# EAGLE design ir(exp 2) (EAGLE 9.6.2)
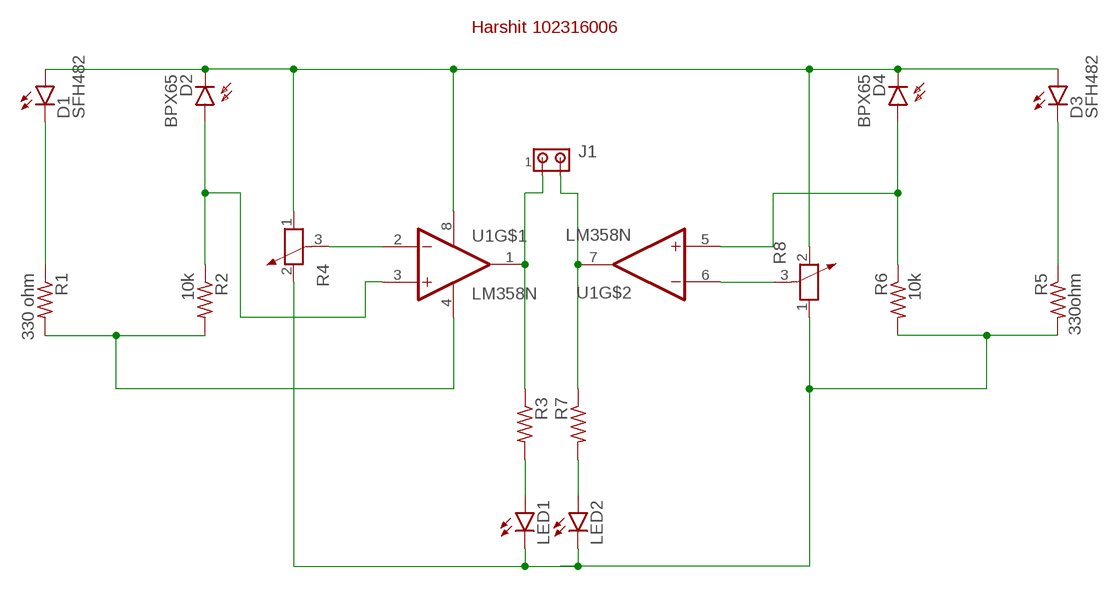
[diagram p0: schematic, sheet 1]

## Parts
D1  SFH482  [SFH482]
D2  BPX65  [BPX65]
D3  SFH482  [SFH482]
D4  BPX65  [BPX65]
J1  MTA02-100  [10X02MTA]
LED1  LED3MM  [LED3MM]
LED2  LED3MM  [LED3MM]
R1  330 ohm  R-US_0204/5  [0204/5]
R2  10k  R-US_0204/5  [0204/5]
R3  R-US_0204/5  [0204/5]
R4  POTENTIOMETER_PT-10  [PT-10]
R5  330ohm  R-US_0204/5  [0204/5]
R6  10k  R-US_0204/5  [0204/5]
R7  R-US_0204/5  [0204/5]
R8  POTENTIOMETER_PT-10  [PT-10]
U1  LM358N  [DIP762W46P254L960H508Q8]

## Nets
N$1: R8.3 U1.6(2IN-)
N$2: D1.K(C) R1.1
N$3: R1.2 R2.2 U1.4(GND)
N$4: D2.A R2.1 U1.3(1IN+)
N$6: LED1.A R3.2
N$7: J1.1 R3.1 U1.1(1OUT)
N$8: R4.3 U1.2(1IN-)
N$9: D1.A D2.K(C) D3.A D4.K(C) R4.1 R8.2 U1.8(VCC)
N$10: D3.K(C) R5.1
N$11: LED1.K(C) LED2.K(C) R4.2 R5.2 R6.2 R8.1
N$12: D4.A R6.1 U1.5(2IN+)
N$14: J1.2 R7.1 U1.7(2OUT)
N$15: LED2.A R7.2

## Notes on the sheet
- Harshit 102316006

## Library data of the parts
D1 D3 = led:SFH482: IR LED
D2 D4 = opto-trans-siemens:BPX65: PHOTO DIODE; MPN: BPX65.; OC_FARNELL: 327451; OC_NEWARK: 06WX2764
J1 = con-amp:MTA02-100: AMP connector
LED1 LED2 = led:LED: LED
R1-R3 R5-R7 = rcl:R-US_: RESISTOR, American symbol; SPICEPREFIX: R
R4 R8 = rcl:POTENTIOMETER_: Potentiometer; SPICEMODEL: POT; SPICEPREFIX: X
U1 = LM358N:LM358N: IC OPAMP GP 2 CIRCUIT 8DIP Check availability; AVAILABILITY: Not in stock; CHECK_PRICES: https://www.snapeda.com/parts/LM358N/Harris/view-part/?ref=eda; DESCRIPTION: General Purpose Amplifier 2 Circuit 8-PDIP; MF: Harris Corporation; MP: LM358N; PACKAGE: None; PRICE: None; SNAPEDA_LINK: https://www.snapeda.com/parts/LM358N/Harris/view-part/?ref=snap

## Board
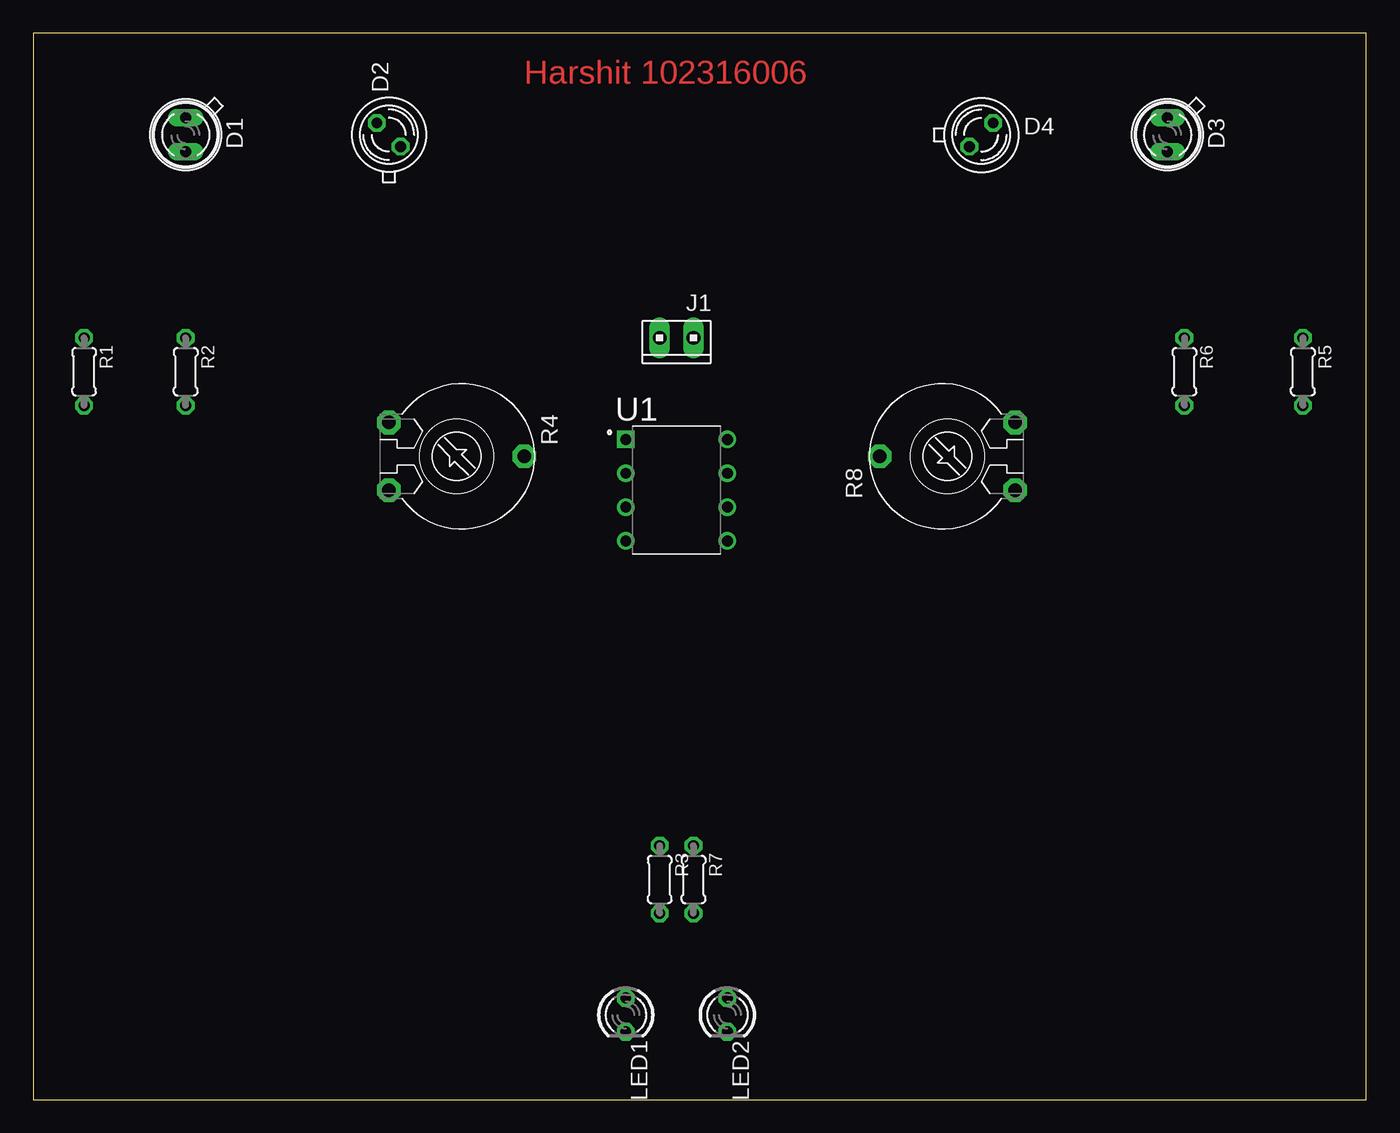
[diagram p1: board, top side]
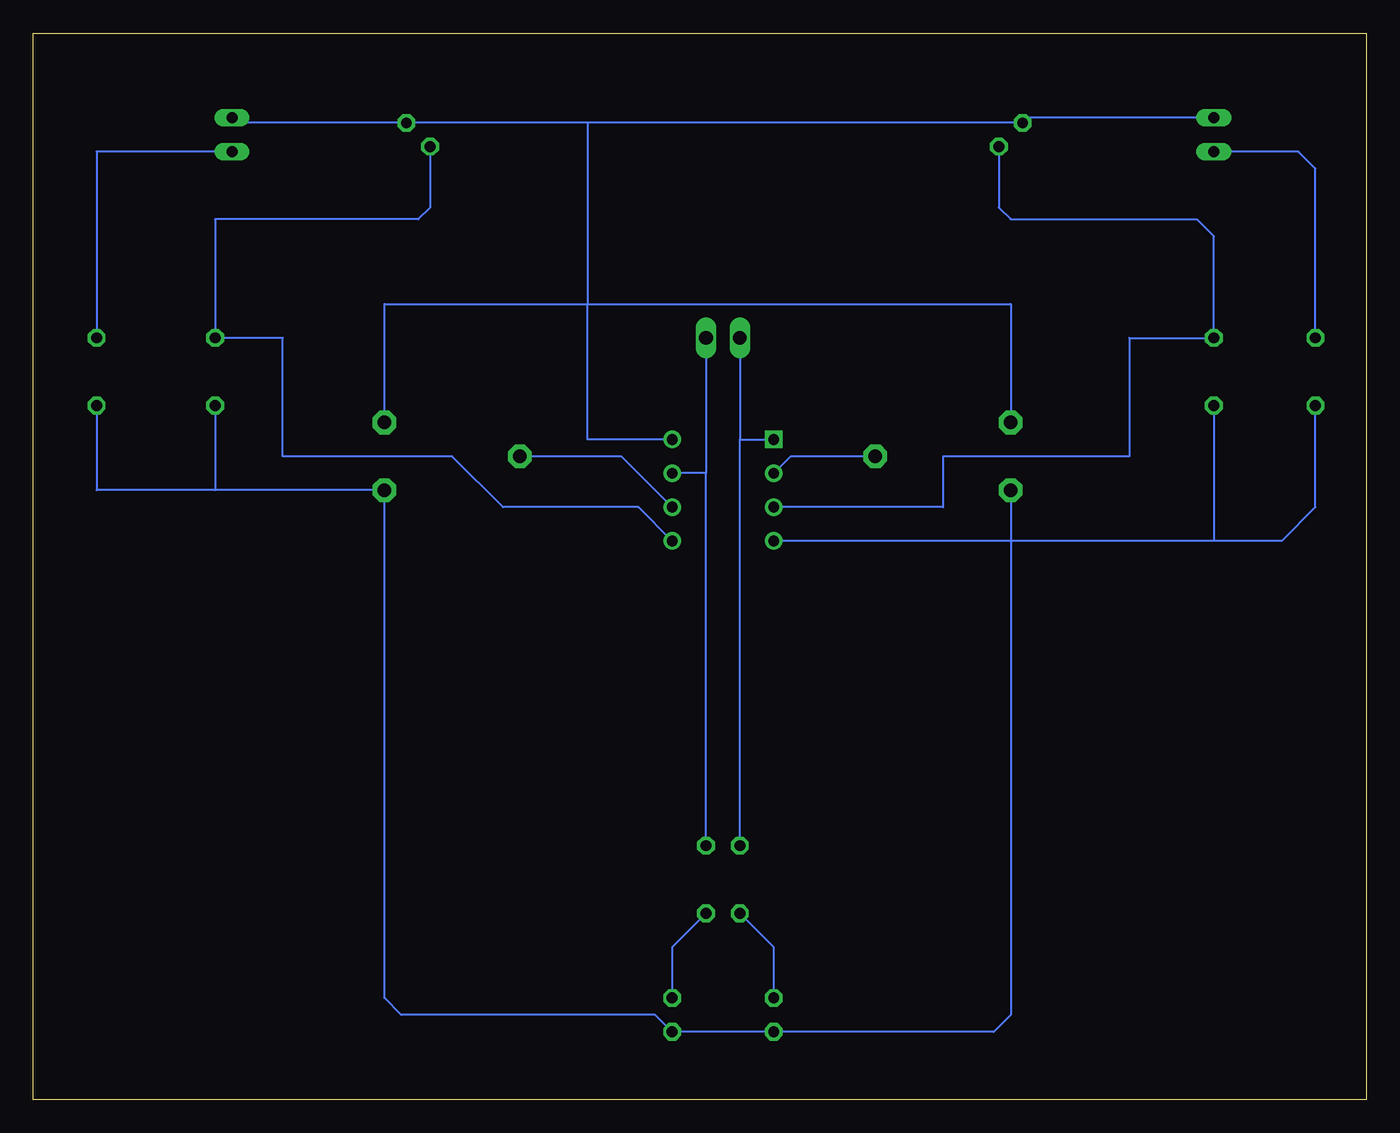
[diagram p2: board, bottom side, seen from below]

Size 100 x 80 mm. Coordinates in mm from the lower left corner, seen from the top.
Outline: 0,0 100,0 100,80 0,80 0,0
Copper layers (1*16): Top 0.035mm / dielectric 1.5mm / Bottom 0.035mm
Design rules "default": minimum track width 6mil, minimum drill 0.35mm, track to track 6mil, track to pad 6mil, pad to pad 6mil, via to via 6mil, smd to smd 6mil, copper to edge 40mil, drill to drill 6mil, minimum pad ring 10mil, minimum via ring 8mil, stop-mask expansion 4mil, vias tented up to drill 0mil, thermal gap 10mil

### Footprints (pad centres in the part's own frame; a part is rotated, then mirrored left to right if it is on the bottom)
SFH482 = drill 0.813 long: A -1.27,0; K 1.27,0
BPX65 = drill 0.813 octagon: A -0.889,-0.889; K 0.889,0.889
10X02MTA = drill 1.016 long: 1 1.27,0; 2 -1.27,0
LED3MM = drill 0.813 octagon: A -1.27,0; K 1.27,0
0204/5 = drill 0.813 octagon: 1 -2.54,0; 2 2.54,0
PT-10 = drill 1.016 pad 1.778 octagon: 1 -2.54,-5.08; 2 2.54,-5.08; 3 0,5.08
DIP762W46P254L960H508Q8 = drill 0.81 pad 1.22 square: 1 -3.81,3.81 | drill 0.81 pad 1.22: 2 -3.81,1.27; 3 -3.81,-1.27; 4 -3.81,-3.81; 5 3.81,-3.81; 6 3.81,-1.27; 7 3.81,1.27; 8 3.81,3.81

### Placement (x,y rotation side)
D1  11.43,72.39 270 top
D2  26.67,72.39 90 top
D3  85.09,72.39 270 top
D4  71.12,72.39 0 top
J1  48.26,57.15 180 top
LED1  44.45,6.35 270 top
LED2  52.07,6.35 270 top
R1  3.81,54.61 270 top
R2  11.43,54.61 270 top
R3  46.99,16.51 270 top
R4  31.75,48.26 270 top
R5  95.25,54.61 270 top
R6  86.36,54.61 270 top
R7  49.53,16.51 270 top
R8  68.58,48.26 90 top
U1  48.26,45.72 0 top

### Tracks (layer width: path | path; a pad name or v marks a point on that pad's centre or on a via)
N$1
  Bottom 0.152: U1.6 55.88,48.26 R8.3
N$2
  Bottom 0.152: R1.1 3.81,69.85 5.08,71.12 D1.K
N$3
  Bottom 0.152: 11.43,41.91 6.35,41.91 3.81,44.45 R1.2 | R2.2 11.43,41.91 | 11.43,41.91 U1.4
N$4
  Bottom 0.152: D2.A 27.56,66.93 26.67,66.04 12.7,66.04 11.43,64.77 R2.1 17.78,57.15 17.78,48.26 31.75,48.26 31.75,44.45 U1.3
N$6
  Bottom 0.152: LED1.A 44.45,11.43 R3.2
N$7
  Bottom 0.152: R3.1 46.99,49.53 | 46.99,49.53 U1.1 | J1.1 46.99,49.53
N$8
  Bottom 0.152: U1.2 43.18,48.26 R4.3
N$9
  Bottom 0.152: D1.A 25.4,73.66 D2.K 58.42,73.28 | 58.42,73.28 D4.K 84.71,73.28 D3.A | R8.2 73.66,59.69 58.42,59.69 | R4.1 26.67,59.69 58.42,59.69 | U1.8 58.42,49.53 58.42,59.69 | 58.42,73.28 58.42,59.69
N$10
  Bottom 0.152: D3.K 95.25,71.12 R5.1
N$11
  Bottom 0.152: R5.2 95.25,45.72 86.36,45.72 | 86.36,45.72 R8.1 73.66,7.62 72.39,6.35 53.34,6.35 LED2.K LED1.K 27.94,5.08 26.67,6.35 R4.2 | R6.2 86.36,45.72
N$12
  Bottom 0.152: D4.A 70.23,66.93 71.12,66.04 86.36,66.04 R6.1 81.28,57.15 81.28,48.26 68.58,48.26 64.77,44.45 54.61,44.45 U1.5
N$14
  Bottom 0.152: 49.15,57.15 J1.2 49.53,46.99 | R7.1 49.53,46.99 | 49.53,46.99 U1.7
N$15
  Bottom 0.152: R7.2 52.07,11.43 LED2.A

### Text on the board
Top: Harshit 102316006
